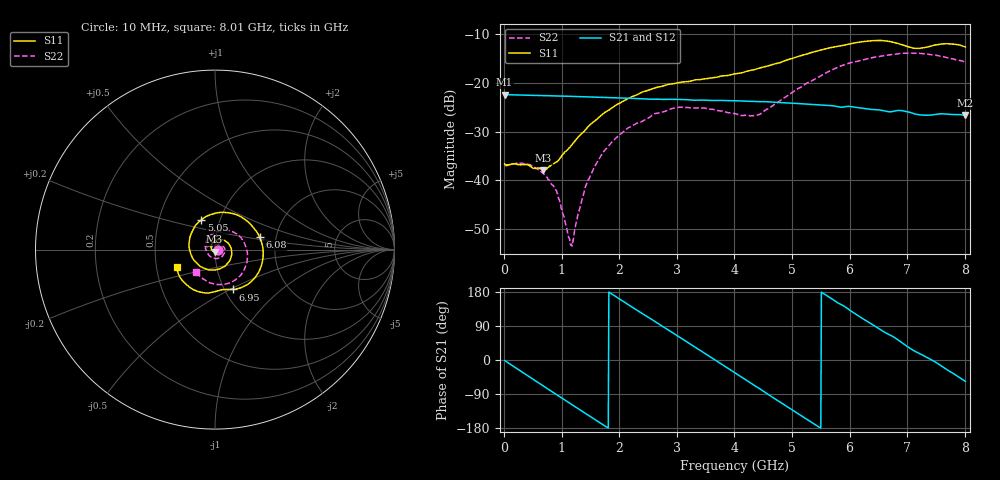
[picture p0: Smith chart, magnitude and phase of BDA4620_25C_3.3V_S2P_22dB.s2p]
!Agilent Technologies,E5071B,MY42404982,A.09.10
!Date: Wed May 06 08:53:32 2026
!Data & Calibration Information:
!Freq	S11:SOLT2(ON)	S21:SOLT2(ON)	S12:SOLT2(ON)	S22:SOLT2(ON)
# Hz S RI R 50
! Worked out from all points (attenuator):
!   801 points, 10 MHz to 8.01 GHz, reference 50 ohm
!   highest |S21| = -22.40 dB at 10 MHz (marker M1); lowest = -26.7 dB at 8.01 GHz (marker M2)
!   lowest |S11| = -38.0 dB at 680 MHz (marker M3), VSWR 1.03, Z = 49.8 - j1.23 ohm
!   |S11| at or under -10 dB: start of sweep to end of sweep
!   |S22| runs from -53.6 to -13.8 dB; largest |S21 - S12| = 0.00036
!   S11 on the Smith chart (normalised r, x): 10 MHz: 1.03, -0.00; 5.05 GHz: 0.82, +0.28; 6.08 GHz: 1.64, +0.25; 6.95 GHz: 1.09, -0.51; 8.01 GHz: 0.64, -0.13
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1e7  0.0147 -0.000978  0.0759 -0.00156  0.076 -0.00164  0.0141 -0.000432
4.1e8  0.00877 -0.0114  0.0562 -0.0494  0.0562 -0.0496  0.0137 -0.00498
6.8e8  -0.0023 -0.0124  0.0275 -0.0689  0.0275 -0.0691  0.00929 -0.0071
9.2e8  -0.014 -0.00667  -0.00269 -0.0735  -0.00276 -0.0736  0.0036 -0.0065
1.16e9  -0.0212 0.00726  -0.0318 -0.0656  -0.0319 -0.0656  -0.0018 -0.00116
1.2e9  -0.0218 0.0101  -0.0362 -0.0631  -0.0363 -0.0631  -0.00239 4.16e-05
1.35e9  -0.0215 0.0213  -0.0509 -0.0514  -0.0508 -0.0515  -0.00394 0.00469
1.53e9  -0.0157 0.0354  -0.0635 -0.0333  -0.0636 -0.0333  -0.00373 0.0115
1.77e9  0.0012 0.0504  -0.0708 -0.00508  -0.0709 -0.00512  0.000586 0.0209
2.14e9  0.0415 0.0546  -0.0591 0.0372  -0.0592 0.0373  0.0168 0.0295
2.68e9  0.0909 0.00505  -0.0068 0.0678  -0.00668 0.0678  0.045 0.0195
3.08e9  0.0832 -0.0593  0.037 0.0565  0.0372 0.0565  0.0558 -0.00771
4.01e9  -0.0842 -0.0914  0.0544 -0.0367  0.0545 -0.0368  -0.0111 -0.0471
4.42e9  -0.1416 -0.00317  0.0176 -0.0618  0.0176 -0.062  -0.0455 -0.0129
5.05e9  -0.0761 0.1658  -0.0446 -0.0427  -0.0447 -0.0428  -0.026 0.0793
5.35e9  0.0192 0.206  -0.0581 -0.015  -0.0582 -0.0151  0.0231 0.1031
6.08e9  0.2483 0.0713  -0.0312 0.0471  -0.0312 0.0473  0.1585 0.0465
6.39e9  0.2645 -0.0653  -0.00371 0.0533  -0.0037 0.0533  0.1808 -0.0215
6.68e9  0.1975 -0.1822  0.0195 0.0466  0.0195 0.0469  0.1712 -0.0914
6.95e9  0.098 -0.222  0.0389 0.0336  0.0389 0.0335  0.1355 -0.1505
7.57e9  -0.0838 -0.2361  0.0468 -0.0111  0.0469 -0.0111  -0.0175 -0.1885
8.01e9  -0.2131 -0.0992  0.0256 -0.0386  0.0256 -0.0387  -0.1036 -0.1272
